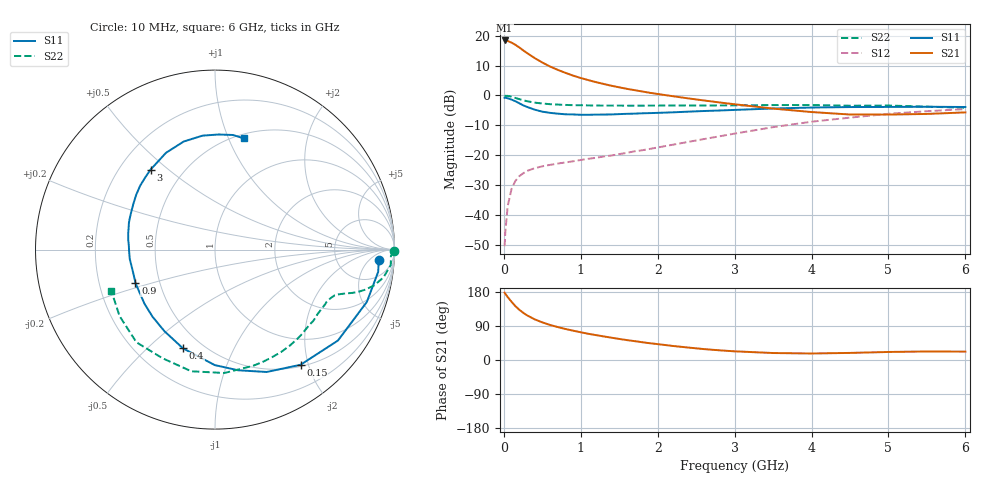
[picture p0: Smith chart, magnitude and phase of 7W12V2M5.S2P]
! Infineon Technologies  Discrete & RF Semiconductors
! BFS17W
! Si NPN RF Bipolar Junction Transistor in SOT323
! VCE = 12 V  IC = 2.5 mA
! Common Emitter S-Parameters:  August  1999
# GHz  S  MA  R  50
!  f  S11  S21  S12  S22
! GHz  MAG  ANG  MAG  ANG  MAG  ANG  MAG  ANG
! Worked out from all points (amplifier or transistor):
!   36 points, 10 MHz to 6 GHz, reference 50 ohm
!   highest |S21| = 18.4 dB at 10 MHz (marker M1)
!   |S21| within 3 dB of that: start of sweep to 235.4 MHz
!   unconditionally stable (mu >= 1): 797.3 MHz to 2.467 GHz; 5.096 GHz to end of sweep
!   at 250 MHz: K = 0.40, MSG = 20.6 dB, |S12| = -26.1 dB
!   at 1.4 GHz: K = 1.24, MAG = 8.7 dB, |S12| = -20.1 dB
!   at 6 GHz: K = 1.06, MAG = -2.1 dB, |S12| = -4.6 dB
!   S11 on the Smith chart (normalised r, x): 10 MHz: 15, -11; 150 MHz: 0.53, -1.87; 400 MHz: 0.39, -0.65; 900 MHz: 0.36, -0.18; 3 GHz: 0.33, +0.44; 6 GHz: 0.54, +1.14
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0.01  0.9144 -3.7  8.316 177.6  0.003 80.2  0.9991 -0.5
0.02  0.9175 -7.8  8.281 174.4  0.0053 89.5  0.9807 -2.0
0.05  0.8949 -19.0  8.145 166.1  0.014 80.9  0.9831 -5.0
0.1  0.852 -36.5  7.652 153.7  0.0272 70.8  0.9513 -9.4
0.15  0.7993 -53.4  7.032 142.1  0.0371 62.3  0.9083 -12.7
0.2  0.7402 -67.1  6.363 132.7  0.0444 57.8  0.8674 -14.9
0.25  0.6844 -79.2  5.702 124.8  0.0496 53.1  0.8304 -16.5
0.3  0.6435 -90.1  5.142 118.1  0.0544 50.7  0.802 -17.5
0.4  0.5783 -108.0  4.223 107.4  0.0605 46.7  0.7582 -18.9
0.5  0.5348 -121.8  3.556 99.3  0.0651 45.7  0.7321 -19.9
0.6  0.5108 -133.0  3.05 92.5  0.0688 46.0  0.7138 -20.9
0.7  0.4953 -142.5  2.68 87.0  0.0724 47.0  0.7028 -22.2
0.9  0.4805 -157.3  2.147 77.4  0.0789 49.7  0.6869 -25.0
1.1  0.4742 -169.3  1.802 69.1  0.087 53.2  0.6805 -28.5
1.3  0.4786 -178.9  1.553 62.1  0.0952 56.7  0.675 -32.3
1.6  0.4922 169.3  1.288 52.5  0.1094 61.7  0.6729 -38.3
2.2  0.5215 150.7  0.969 37.0  0.1499 69.8  0.6781 -52.0
3  0.5721 128.9  0.711 22.9  0.2296 72.7  0.6813 -71.8
3.5  0.6044 116.9  0.602 18.4  0.2944 70.5  0.6895 -85.6
4.5  0.6387 96.2  0.479 18.7  0.4251 59.1  0.6722 -115.9
5.5  0.6463 81.1  0.49 22.5  0.5444 45.4  0.648 -145.1
6  0.64 75.4  0.52 22.1  0.5911 38.5  0.622 -158.2
